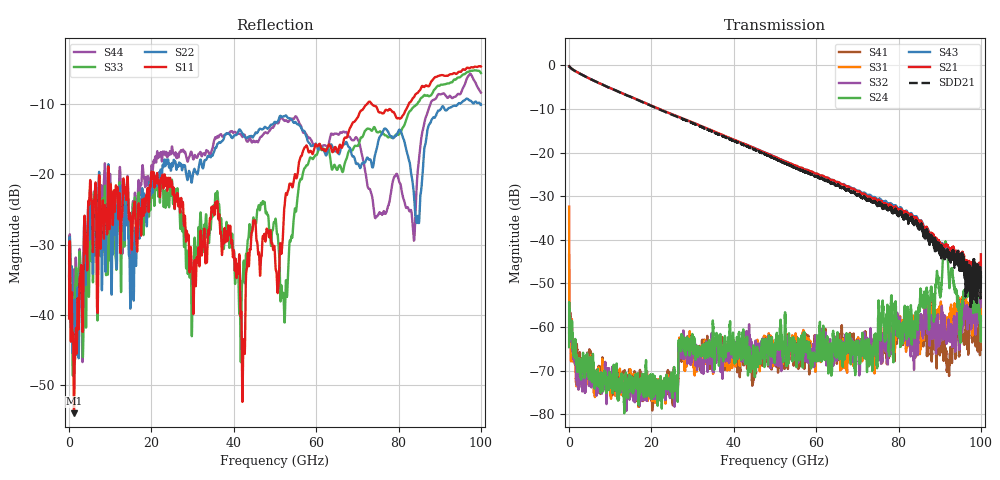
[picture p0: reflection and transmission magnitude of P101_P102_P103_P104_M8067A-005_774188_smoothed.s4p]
!Keysight Technologies PLTS 2021(64 bit), Build 20210202.1
!S11 smoothed in format LOGMAG, average points = 21
!S12 smoothed in format LOGMAG, average points = 21
!S13 smoothed in format LOGMAG, average points = 21
!S14 smoothed in format LOGMAG, average points = 21
!S21 smoothed in format LOGMAG, average points = 21
!S22 smoothed in format LOGMAG, average points = 21
!S23 smoothed in format LOGMAG, average points = 21
!S24 smoothed in format LOGMAG, average points = 21
!S31 smoothed in format LOGMAG, average points = 21
!S32 smoothed in format LOGMAG, average points = 21
!S33 smoothed in format LOGMAG, average points = 21
!S34 smoothed in format LOGMAG, average points = 21
!S41 smoothed in format LOGMAG, average points = 21
!S42 smoothed in format LOGMAG, average points = 21
!S43 smoothed in format LOGMAG, average points = 21
!S44 smoothed in format LOGMAG, average points = 21
!$DUT_CFG_DESC: Default 4-Port Configuration
!$NUMBER_PORTS: 4
!$DIFF_PORT_MAP: 1|2P|2|2P|0|UC|0|UC|
!$PORT_MAP: 1|1|<<<<<<|2|2|>>>>>>|3|3|<<<<<<|4|4|>>>>>>|
!Date: Monday, December 04, 2023, 05:49:59
!S4P File: Measurements: <S11,S12,S13,S14>,
!<S21,S22,S23,S24>,
!<S31,S32,S33,S34>,
!<S41,S42,S43,S44>:
# MHz S  RI  R 50
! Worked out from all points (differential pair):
!   10000 points, 10 MHz to 100 GHz, reference 50 ohm
!   strongest paths, dB at 10 MHz, 25.01 GHz, 50.01 GHz, 75.01 GHz, 100 GHz:
!     S21: -0.2, -11.2, -21.0, -30.9, -43.3
!     S43: -0.3, -11.3, -21.0, -30.7, -47.6
!     S24: -64.6, -72.8, -66.6, -60.5, -58.8
!     S32: -61.4, -72.8, -66.9, -62.9, -48.9
!     S31: -32.4, -72.6, -64.4, -63.5, -58.5
!     S41: -43.5, -73.7, -66.1, -65.0, -65.2
!   taken as a pair (ports 1,3 in; 2,4 out), SDD21 dB: -0.2, -11.3, -21.5, -32.2, -48.1
!   lowest |S11| = -54.0 dB at 1.2 GHz (marker M1), VSWR 1.00, Z = 50.1 - j0.164 ohm
!   |S11| at or under -10 dB: start of sweep to 72.41 GHz; 73.46 GHz to 82.49 GHz (9.033 GHz wide, 11.6 % of centre)
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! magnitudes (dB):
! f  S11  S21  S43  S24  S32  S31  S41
! 10 MHz  -40.5  -0.2  -0.3  -64.6  -61.4  -32.4  -43.5
! 1.2 GHz  -54.0  -1.2  -1.2  -66.8  -66.4  -66.6  -64.7
! 5.1 GHz  -20.9  -3.1  -3.1  -68.7  -68.5  -69.4  -68.7
! 42.31 GHz  -44.6  -17.9  -18.0  -61.1  -66.1  -67.1  -66.4
! 57.28 GHz  -16.2  -23.9  -23.9  -63.8  -67.9  -63.7  -64.7
! 91.35 GHz  -6.0  -41.6  -42.4  -40.4  -61.1  -58.6  -67.5
! 100 GHz  -4.7  -43.3  -47.6  -58.8  -48.9  -58.5  -65.2
